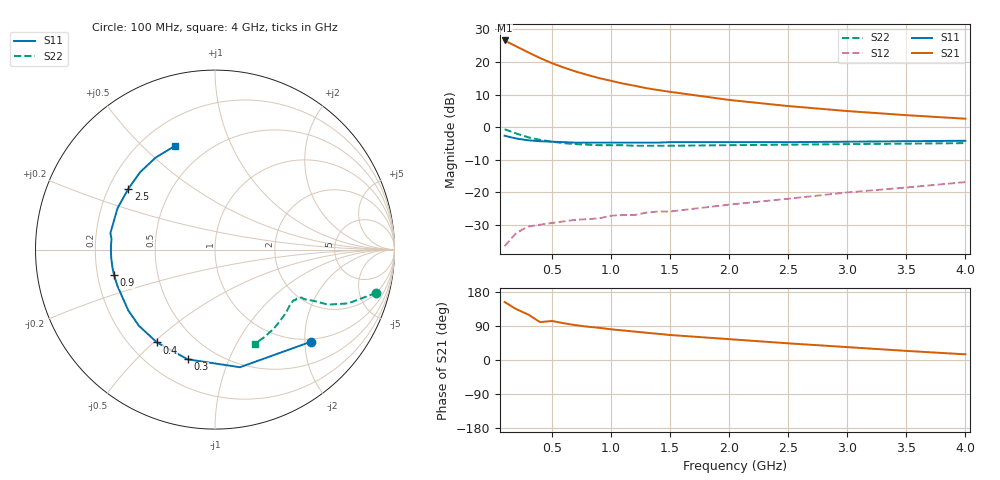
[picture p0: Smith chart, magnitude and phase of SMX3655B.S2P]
! HSMX-3655  COMMON EMITTER
! Vce=10v Ic=10ma
# ghz s ma r 50
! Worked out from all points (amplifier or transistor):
!   20 points, 100 MHz to 4 GHz, reference 50 ohm
!   highest |S21| = 26.6 dB at 100 MHz (marker M1)
!   |S21| within 3 dB of that: start of sweep to 263.7 MHz
!   unconditionally stable (mu >= 1): 1.13 GHz to 3.253 GHz
!   at 400 MHz: K = 0.54, MSG = 25.6 dB, |S12| = -29.9 dB
!   at 1.1 GHz: K = 0.97, MSG = 20.2 dB, |S12| = -26.9 dB
!   at 4 GHz: K = 0.87, MSG = 9.7 dB, |S12| = -16.8 dB
!   lowest NFmin = 1.40 dB at 500 MHz
!   S11 on the Smith chart (normalised r, x): 100 MHz: 0.94, -2.13; 300 MHz: 0.35, -0.72; 400 MHz: 0.31, -0.51; 900 MHz: 0.27, -0.11; 2.5 GHz: 0.28, +0.29; 4 GHz: 0.34, +0.63
0.1  0.74 -44.0  21.39 153.0  0.015 65.0  0.93 -15.0
0.2  0.67 -78.0  17.29 134.0  0.024 55.0  0.8 -22.0
0.3  0.63 -104.0  14.04 120.0  0.03 48.0  0.7 -26.0
0.4  0.61 -122.0  11.49 100.0  0.032 44.0  0.64 -27.0
0.5  0.6 -135.0  9.6 103.0  0.034 43.0  0.6 -28.0
0.6  0.59 -145.0  8.23 97.0  0.036 42.0  0.57 -29.0
0.7  0.58 -153.0  7.16 92.0  0.038 43.0  0.55 -29.0
0.8  0.58 -160.0  6.34 88.0  0.039 45.0  0.54 -30.0
0.9  0.58 -166.0  5.66 85.0  0.04 45.0  0.53 -31.0
1  0.58 -170.0  5.15 81.0  0.044 47.0  0.53 -31.0
1.1  0.58 -175.0  4.67 78.0  0.045 45.0  0.53 -32.0
1.2  0.58 -179.0  4.33 75.0  0.045 50.0  0.52 -33.0
1.3  0.58 178.0  3.97 72.0  0.049 51.0  0.52 -34.0
1.4  0.58 174.0  3.71 69.0  0.051 52.0  0.52 -36.0
1.5  0.59 171.0  3.49 66.0  0.051 55.0  0.52 -37.0
2  0.59 157.0  2.62 55.0  0.065 60.0  0.53 -42.0
2.5  0.59 145.0  2.11 44.0  0.08 64.0  0.54 -49.0
3  0.6 134.0  1.77 34.0  0.1 63.0  0.55 -54.0
3.5  0.61 123.0  1.53 24.0  0.119 64.0  0.56 -61.0
4  0.62 111.0  1.35 15.0  0.144 62.0  0.57 -67.0
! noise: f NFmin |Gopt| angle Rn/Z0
0.5  1.4  0.1  69  0.26
1  1.5  0.2  118  0.02
1.5  1.8  0.41  148  0.06
2  2  0.35  178  0.18
